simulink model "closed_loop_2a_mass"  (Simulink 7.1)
settings: Solver=FixedStepDiscrete  StartTime=0.0  StopTime=Tend  FixedStep=Ts  MaxStep=Ts  MinStep=Ts/10  RelTol=1e-4
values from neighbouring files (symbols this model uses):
  Kt = 0.06    [lame_dat.m]
  L1 = 0.040    (= 0.04)    [lame_dat.m]
  L3 = 0.100    (= 0.1)    [lame_dat.m]
  Ts = 100e-6    (= 0.0001)    [lame_main.m]
libraries: powerlib_extras x1, cstblocks x1

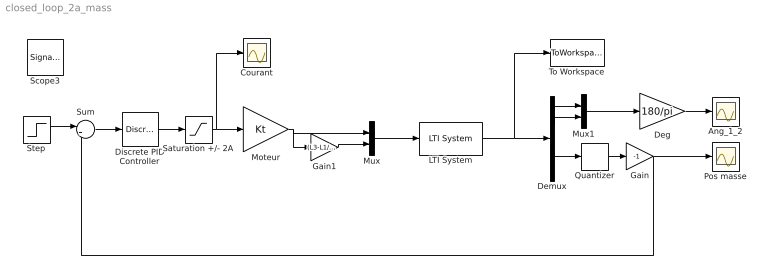
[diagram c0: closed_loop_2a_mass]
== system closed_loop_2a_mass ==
  Ang_1_2 : Scope
  Courant : Scope
  Deg : Gain  Gain=180/pi  ParameterDataType=fixdt(1, 16)  ParameterScaling=2^0  OutDataType=fixdt(1, 16)  OutScaling=2^0
  Demux : Demux  Outputs=5
  Discrete PID Controller : powerlib_extras/Discrete  Control Blocks/Discrete PID Controller  DialogController=POWERSYS.PowerSysDialog  SystemSampleTime=-1  Kp=150  Ki=2000  Kd=0.4  TcD=Ts  Par_Limits="[1    -1]"  Init=0  Ts=Ts
  Gain : Gain  Gain=-1  ParameterDataType=sfix(16)  ParameterScaling=2^0  OutDataType=sfix(16)  OutScaling=2^0
  Gain1 : Gain  Gain=(L3-L1/2)/L1/2  ParameterDataType=sfix(16)  ParameterScaling=2^0  OutDataType=sfix(16)  OutScaling=2^0
  LTI System : cstblocks/LTI System  SystemSampleTime=-1  sys=sysd  IC=[]
  Moteur : Gain  Gain=Kt  ParameterDataType=sfix(16)  ParameterScaling=2^0  OutDataType=sfix(16)  OutScaling=2^0
  Mux : Mux  Inputs=2
  Mux1 : Mux  Inputs=2
  Pos masse : Scope
  Quantizer : Quantizer  QuantizationInterval=10e-6
  Saturation +/- 2A : Saturate  UpperLimit=2  LowerLimit=-2  OutDataType=sfix(16)  OutScaling=2^0
  Step : Step  Time=0  After=0.001  SampleTime=0
  Sum : Sum  Inputs=|+-  OutDataType=sfix(16)  OutScaling=2^0
  To Workspace : ToWorkspace  VariableName=y_sim_out  SampleTime=-1  SaveFormat=Structure With Time
  Scope3 : SignalViewerScope  IOType=viewer  RefreshTime=0.035000
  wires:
  Deg/1 -> Ang_1_2/1
  LTI System/1 -> Demux/1, To Workspace/1
  Moteur/1 -> Mux/1, Gain1/1
  Mux/1 -> LTI System/1
  Step/1 -> Sum/1
  Sum/1 -> Discrete PID Controller/1
  Discrete PID Controller/1 -> Saturation +/- 2A/1
  Saturation +/- 2A/1 -> Moteur/1, Courant/1
  Demux/4 -> Quantizer/1
  Quantizer/1 -> Gain/1
  Demux/1 -> Mux1/1
  Demux/2 -> Mux1/2
  Mux1/1 -> Deg/1
  Gain1/1 -> Mux/2
  Gain/1 -> Pos masse/1, Sum/2
